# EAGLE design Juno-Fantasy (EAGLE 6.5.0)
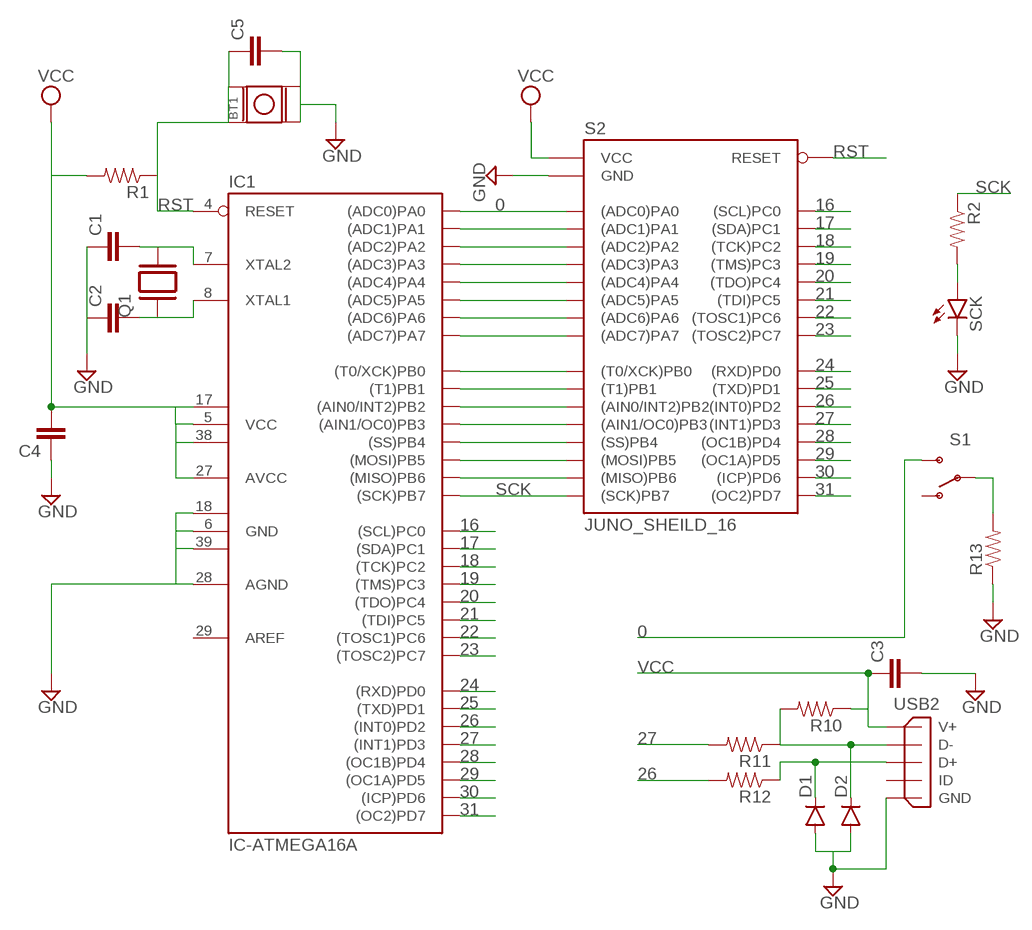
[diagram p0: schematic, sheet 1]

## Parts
BT1  BUTTON-4X4-SMD  [BUT-SMD-4X4]
C1  CAP-SMD-0805  [0805]
C2  CAP-SMD-0805  [0805]
C3  CAP-SMD-0805  [0805]
C4  CAP-SMD-0805  [0805]
C5  CAP-SMD-0805  [0805]
D1  DIODE-SOD-1206  [SOD-1206]
D2  DIODE-SOD-1206  [SOD-1206]
IC1  IC-ATMEGA16A  [TQFP44]
Q1  CRYSTAL-2*6-TH  [CRYSTAL-2*6MM-TH]
R1  RESISTOR-SMD-0805  [0805-R]
R2  RESISTOR-SMD-0805  [0805-R]
R10  RESISTOR-SMD-0805  [0805-R]
R11  RESISTOR-SMD-0805  [0805-R]
R12  RESISTOR-SMD-0805  [0805-R]
R13  RESISTOR-SMD-0805  [0805-R]
S1  SPDT-SMALL-MSK-12C01  [SPDT-SMD]
S2  JUNO_SHEILD_16  [JUNO_SHEILD_16]
SCK  LED-SMD-0805  [LED-0805]
USB2  USB-MICRO  [USB-MICRO]

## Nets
0: IC1.37((ADC0)PA0) S1.1(OFF) S2.A0((ADC0)PA0) S2.A0-((ADC0)PA0)
16: IC1.19((SCL)PC0) S2.C0((SCL)PC0) S2.C0-((SCL)PC0)
17: IC1.20((SDA)PC1) S2.C1((SDA)PC1) S2.C1-((SDA)PC1)
18: IC1.21((TCK)PC2) S2.C2((TCK)PC2) S2.C2-((TCK)PC2)
19: IC1.22((TMS)PC3) S2.C3((TMS)PC3) S2.C3-((TMS)PC3)
20: IC1.23((TDO)PC4) S2.C4((TDO)PC4) S2.C4-((TDO)PC4)
21: IC1.24((TDI)PC5) S2.C5((TDI)PC5) S2.C5-((TDI)PC5)
22: IC1.25((TOSC1)PC6) S2.C6((TOSC1)PC6) S2.C6-((TOSC1)PC6)
23: IC1.26((TOSC2)PC7) S2.C7((TOSC2)PC7) S2.C7-((TOSC2)PC7)
24: IC1.9((RXD)PD0) S2.D0((RXD)PD0) S2.D0-((RXD)PD0)
25: IC1.10((TXD)PD1) S2.D1((TXD)PD1) S2.D1-((TXD)PD1)
26: IC1.11((INT0)PD2) R12.2 S2.D2((INT0)PD2) S2.D2-((INT0)PD2)
27: IC1.12((INT1)PD3) R11.2 S2.D3((INT1)PD3) S2.D3-((INT1)PD3)
28: IC1.13((OC1B)PD4) S2.D4((OC1B)PD4) S2.D4-((OC1B)PD4)
29: IC1.14((OC1A)PD5) S2.D5((OC1A)PD5) S2.D5-((OC1A)PD5)
30: IC1.15((ICP)PD6) S2.D6((ICP)PD6) S2.D6-((ICP)PD6)
31: IC1.16((OC2)PD7) S2.D7((OC2)PD7) S2.D7-((OC2)PD7)
GND: BT1.A0 BT1.A1 C1.1 C2.1 C3.2 C4.1 C5.2 D1.A D2.A IC1.6(GND) IC1.18(GND1) IC1.28(AGND) IC1.39(GND2) R13.1 S2.GND1(GND) S2.GND2(GND) S2.GND3(GND) SCK.C USB2.GND
N$1: C1.2 IC1.7(XTAL2) Q1.P$2
N$2: C2.2 IC1.8(XTAL1) Q1.P$1
N$3: R13.2 S1.2(MID)
N$4: IC1.36((ADC1)PA1) S2.A1((ADC1)PA1) S2.A1-((ADC1)PA1)
N$5: IC1.35((ADC2)PA2) S2.A2((ADC2)PA2) S2.A2-((ADC2)PA2)
N$6: IC1.34((ADC3)PA3) S2.A3((ADC3)PA3) S2.A3-((ADC3)PA3)
N$7: IC1.33((ADC4)PA4) S2.A4((ADC4)PA4) S2.A4-((ADC4)PA4)
N$8: IC1.32((ADC5)PA5) S2.A5((ADC5)PA5) S2.A5-((ADC5)PA5)
N$9: IC1.31((ADC6)PA6) S2.A6((ADC6)PA6) S2.A6-((ADC6)PA6)
N$10: IC1.30((ADC7)PA7) S2.A7((ADC7)PA7) S2.A7-((ADC7)PA7)
N$12: IC1.40((T0/XCK)PB0) S2.B0((T0/XCK)PB0) S2.B0-((T0/XCK)PB0)
N$13: IC1.41((T1)PB1) S2.B1((T1)PB1) S2.B1-((T1)PB1)
N$14: IC1.42((AIN0/INT2)PB2) S2.B2((AIN0/INT2)PB2) S2.B2-((AIN0/INT2)PB2)
N$15: IC1.43((AIN1/OC0)PB3) S2.B3((AIN1/OC0)PB3) S2.B3-((AIN1/OC0)PB3)
N$16: IC1.44((SS)PB4) S2.B4((SS)PB4) S2.B4-((SS)PB4)
N$17: IC1.1((MOSI)PB5) S2.B5((MOSI)PB5) S2.B5-((MOSI)PB5) S2.MOSI((MOSI)PB5)
N$18: IC1.2((MISO)PB6) S2.B6((MISO)PB6) S2.B6-((MISO)PB6) S2.MISO((MISO)PB6)
N$20: R2.2 SCK.A
N$29: D2.C R10.2 R11.1 USB2.D-
N$30: D1.C R12.1 USB2.D+
RST: BT1.B1(B0) BT1.B2(B1) C5.1 IC1.4(RESET) R1.1 S2.RST1(RESET) S2.RST2(RESET)
SCK: IC1.3((SCK)PB7) R2.1 S2.B7((SCK)PB7) S2.B7-((SCK)PB7) S2.SCK((SCK)PB7)
VCC: C3.1 C4.2 IC1.5(VCC) IC1.17(VCC1) IC1.27(AVCC) IC1.38(VCC2) R1.2 R10.1 S2.VCC1(VCC) S2.VCC2(VCC) S2.VCC3(VCC) USB2.V+
Unconnected: S1.3(ON) USB2.ID

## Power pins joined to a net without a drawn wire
AREF: IC1.29(AREF)

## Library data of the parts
BT1 = My Eagle lbr:BUTTON
C1-C5 = My Eagle lbr:CAP-SMD
D1 D2 = My Eagle lbr:DIODE: Diode
IC1 = My Eagle lbr:IC-ATMEGA16: MICROCONTROLLER 16 Kbytes FLASH 1 kbytes SRAM 512 bytes EEPROM USART 8-channel 10 bit ADC
Q1 = My Eagle lbr:CRYSTAL: CRYSTAL
R1 R2 R10-R13 = My Eagle lbr:RESISTOR-SMD
S1 = My Eagle lbr:SPDT-SMALL: SPDT-Switch
S2 = My Eagle lbr:JUNO_SHEILD_16
SCK = My Eagle lbr:LED-SMD
USB2 = My Eagle lbr:USB

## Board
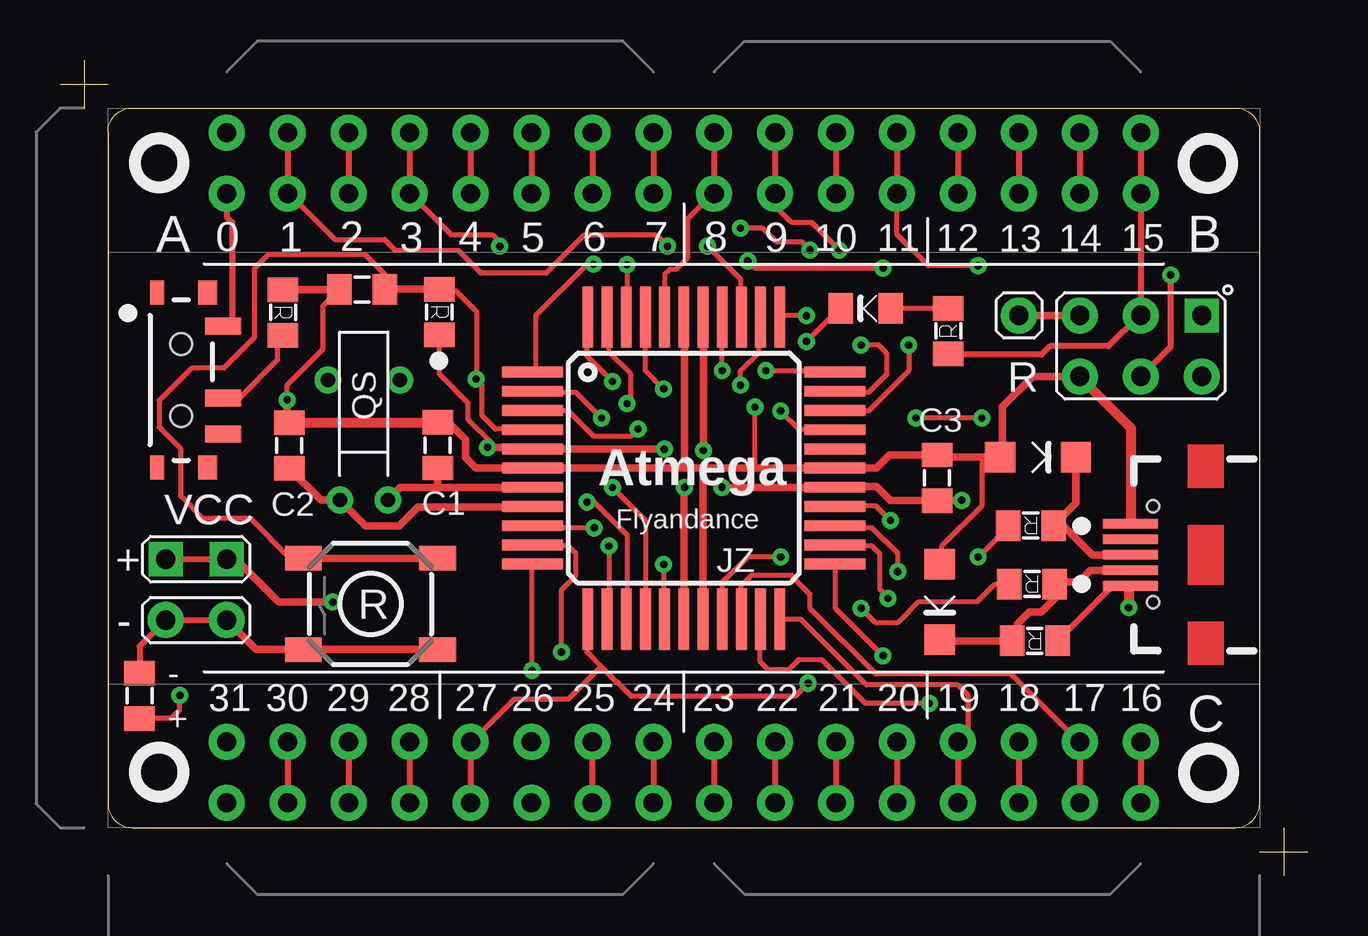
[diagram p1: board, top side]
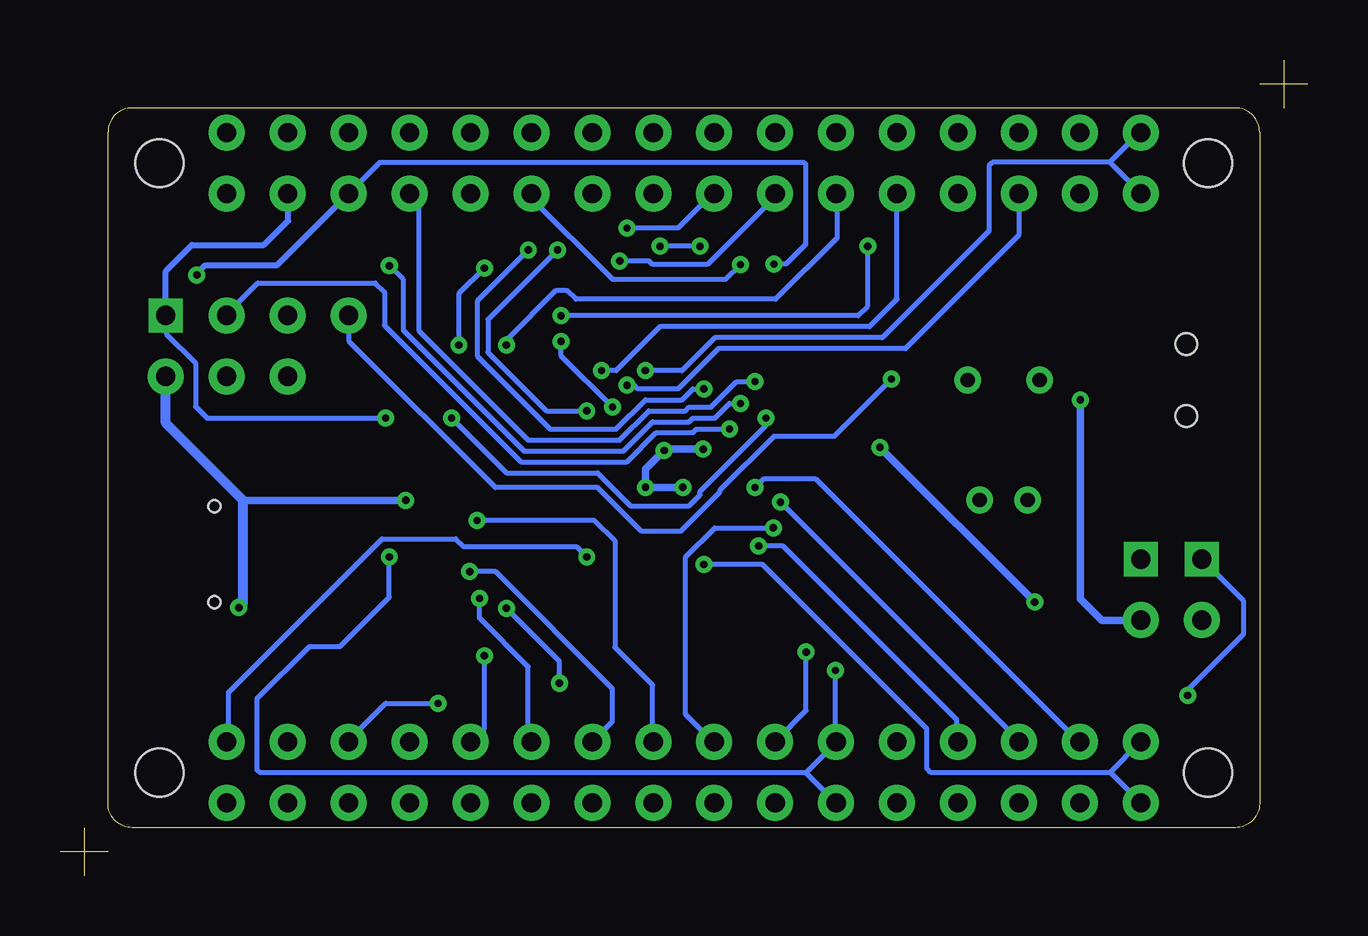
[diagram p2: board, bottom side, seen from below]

Size 52 x 34 mm. Coordinates in mm from the lower left corner, seen from the top.
Outline: 0,33 2,33
Outline: 1,34 1,32
Outline: 50,1 52,1
Outline: 51,2 51,0
Outline: 2,3 arc90 3,2 49,2 arc90 50,3 50,31 arc90 49,32 3,32 arc90 2,31 2,3
Copper layers (1*16): Top 0.035mm / dielectric 1.5mm / Bottom 0.035mm
Design rules "6mm-15mil *": minimum track width 8mil, minimum drill 0.3mm, track to track 6mil, track to pad 15mil, pad to pad 15mil, via to via 10mil, smd to smd 6mil, copper to edge 10mil, drill to drill 6mil, minimum pad ring 10mil, minimum via ring 8mil, stop-mask expansion 1mil, vias tented up to drill 0.4mm, thermal gap 10mil

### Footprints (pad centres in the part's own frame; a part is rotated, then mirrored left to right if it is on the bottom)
BUT-SMD-4X4 = smd 1.524 x 1.016: A0 -2.794,1.905; A1 2.794,1.905; B1 -2.794,-1.905; B2 2.794,-1.905
0805 = smd 1.016 x 1.27: 1 -0.95,0; 2 0.95,0
SOD-1206 = smd 1.27 x 1.27: A 1.575,0; C -1.575,0
TQFP44 = smd 2.55 x 0.45: 1 -6.3,4; 2 -6.3,3.2; 3 -6.3,2.4; 4 -6.3,1.6; 5 -6.3,0.8; 6 -6.3,0; 7 -6.3,-0.8; 8 -6.3,-1.6; 9 -6.3,-2.4; 10 -6.3,-3.2; 11 -6.3,-4; 23 6.3,-4; 24 6.3,-3.2; 25 6.3,-2.4; 26 6.3,-1.6; 27 6.3,-0.8; 28 6.3,0; 29 6.3,0.8; 30 6.3,1.6; 31 6.3,2.4; 32 6.3,3.2; 33 6.3,4 | smd 0.45 x 2.55: 12 -4,-6.3; 13 -3.2,-6.3; 14 -2.4,-6.3; 15 -1.6,-6.3; 16 -0.8,-6.3; 17 0,-6.3; 18 0.8,-6.3; 19 1.6,-6.3; 20 2.4,-6.3; 21 3.2,-6.3; 22 4,-6.3; 34 4,6.3; 35 3.2,6.3; 36 2.4,6.3; 37 1.6,6.3; 38 0.8,6.3; 39 0,6.3; 40 -0.8,6.3; 41 -1.6,6.3; 42 -2.4,6.3; 43 -3.2,6.3; 44 -4,6.3
CRYSTAL-2*6MM-TH = drill 0.6 pad 1: NC1 -1.5,5; NC2 1.5,5 | drill 0.6: P$1 -1,0; P$2 1,0
0805-R = smd 1.016 x 1.27: 1 -0.95,0; 2 0.95,0
SPDT-SMD = smd 1.5 x 0.7: 1 1.75,2.25; 2 1.75,-0.75; 3 1.75,-2.25 | smd 0.6 x 1: GND5 -1,-3.65; GND7 -1,3.65 | smd 0.8 x 1: GND6 1.1,-3.65; GND8 1.1,3.65 | hole 0.9: 0,-1.5; 0,1.5
JUNO_SHEILD_16 = drill 0.8 pad 1.5: A0 -19.05,13.97; A0- -19.05,11.43; A1 -16.51,13.97; A1- -16.51,11.43; A2 -13.97,13.97; A2- -13.97,11.43; A3 -11.43,13.97; A3- -11.43,11.43; A4 -8.89,13.97; A4- -8.89,11.43; A5 -6.35,13.97; A5- -6.35,11.43; A6 -3.81,13.97; A6- -3.81,11.43; A7 -1.27,13.97; A7- -1.27,11.43; B0 1.27,13.97; B0- 1.27,11.43; B1 3.81,13.97; B1- 3.81,11.43; B2 6.35,13.97; B2- 6.35,11.43; B3 8.89,13.97; B3- 8.89,11.43; B4 11.43,13.97; B4- 11.43,11.43; B5 13.97,13.97; B5- 13.97,11.43; B6 16.51,13.97; B6- 16.51,11.43; B7 19.05,13.97; B7- 19.05,11.43; C0 19.05,-13.97; C0- 19.05,-11.43; C1 16.51,-13.97; C1- 16.51,-11.43; C2 13.97,-13.97; C2- 13.97,-11.43; C3 11.43,-13.97; C3- 11.43,-11.43; C4 8.89,-13.97; C4- 8.89,-11.43; C5 6.35,-13.97; C5- 6.35,-11.43; C6 3.81,-13.97; C6- 3.81,-11.43; C7 1.27,-13.97; C7- 1.27,-11.43; D0 -1.27,-13.97; D0- -1.27,-11.43; D1 -3.81,-13.97; D1- -3.81,-11.43; D2 -6.35,-13.97; D2- -6.35,-11.43; D3 -8.89,-13.97; D3- -8.89,-11.43; D4 -11.43,-13.97; D4- -11.43,-11.43; D5 -13.97,-13.97; D5- -13.97,-11.43; D6 -16.51,-13.97; D6- -16.51,-11.43; D7 -19.05,-13.97; D7- -19.05,-11.43; GND1 -21.59,-6.35; GND2 -19.05,-6.35; GND3 16.51,3.81; MOSI 19.05,3.81; RST1 16.51,6.35; RST2 13.97,6.35; SCK 19.05,6.35; VCC3 21.59,3.81 | drill 0.8 pad 1.422 square: MISO 21.59,6.35; VCC1 -21.59,-3.81; VCC2 -19.05,-3.81 | hole 2: -21.86,12.7; 21.86,12.7; 21.86,-12.7; -21.86,-12.7
LED-0805 = smd 1.016 x 1.27: A -1.052,0; C 1.026,0
USB-MICRO = smd 2.3 x 0.4: D+ 1.65,0.016; D- 1.65,0.666; GND 1.65,-1.284; ID 1.65,-0.634; V+ 1.65,1.316 | hole 0.5: 0.708,2; 0.708,-2

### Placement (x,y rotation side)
BT1  12.94,11.32 180 top
C1  15.74,17.94 270 top
C2  9.56,17.93 270 top
C3  36.56,16.58 90 top
C4  3.32,7.5 270 top
C5  12.59,24.43 180 top
D1  40.77,17.44 180 top
D2  36.67,11.4 90 top
IC1  26,16.98 0 top
Q1  12.66,15.66 0 top
R1  15.81,23.49 270 top
R2  37.03,22.7 90 top
R10  40.63,9.78 180 top
R11  40.51,12.15 180 top
R12  40.46,14.59 180 top
R13  9.3,23.47 270 top
S1  5.05,20.66 0 top
S2  26,17 0 top
SCK  33.57,23.64 180 top
USB2  46.27,13.39 180 top

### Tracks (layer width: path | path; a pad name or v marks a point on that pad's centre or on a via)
0  (via drill 0.3)
  Top 0.203: v27.6,21.05 27.6,23.18 IC1.37
  Top 0.254: S2.A0- 6.95,27.45 7.18,27.22 7.18,22.91 S1.1
  Top 0.305: S1.1
  Bottom 0.203: v27.6,21.05 26.08,21.05 24.71,22.42 17.72,22.42 13.28,26.87 13.28,29.58 13.12,29.74 8.25,29.74 | 8.25,29.74 7.03,30.96 S2.A0 | 8.25,29.74 S2.A0-
16  (via drill 0.3)
  Top 0.203: v30.04,13.28 28.67,13.28 27.6,12.21 IC1.19
  Top 0.254: S2.C0- S2.C0
  Bottom 0.203: S2.C0- 44.98,5.66 44.98,7.64 38.58,14.04 35.5,14.04 35.17,13.71 30.47,13.71 v30.04,13.28
17
  Top 0.203: IC1.20 28.36,10.69 28.36,12.06 28.82,12.52 30.5,12.52 30.5,12.49 31.26,11.73 31.26,11.14 34,8.4 39.64,8.4 42.39,5.66 S2.C1-
  Top 0.254: S2.C1- S2.C1
18  (via drill 0.3)
  Top 0.203: 29.28,10.53 IC1.21 29.18,10.66 29.18,8.93 29.53,8.58 30.37,8.58 30.78,8.98 31.77,8.98 33.57,7.18 v36.24,7.18
  Top 0.254: S2.C2- S2.C2
  Bottom 0.203: v36.24,7.18 38.42,7.18 39.95,5.66 S2.C2-
19
  Top 0.203: 30.04,10.53 IC1.22 30.88,10.69 33.62,7.94 37.43,7.94 37.84,7.54 37.84,5.98 S2.C3- 37.36,5.66
  Top 0.254: S2.C3- S2.C3
20  (via drill 0.3)
  Top 0.203: v34.31,9.16 32.33,11.14 32.33,12.97 IC1.23
  Top 0.254: S2.C4- S2.C4
  Bottom 0.203: v34.31,9.16 34.31,6.12 34.77,5.66 S2.C4-
21  (via drill 0.3)
  Top 0.203: IC1.24 32.33,13.73 33.85,13.73 34.16,13.43 34.16,11.96 34.51,11.6 v34.51,11.55
  Top 0.254: S2.C5- S2.C5
  Bottom 0.203: S2.C5- 32.48,5.66 32.48,8.71 34.51,10.74 v34.51,11.55
22  (via drill 0.3)
  Top 0.203: v34.92,12.67 34.92,13.43 33.85,14.5 32.33,14.5 IC1.25
  Top 0.254: S2.C6- S2.C6
  Bottom 0.203: v34.92,12.67 33.85,12.67 28.98,7.79 28.98,6.42 29.74,5.66 S2.C6-
23  (via drill 0.3)
  Top 0.203: v34.61,14.8 34,15.41 32.33,15.41 IC1.26
  Top 0.254: S2.C7- S2.C7
  Bottom 0.203: v34.61,14.8 29.71,14.8 28.87,13.96 28.87,9.52 27.3,7.94 27.3,5.66 S2.C7-
24  (via drill 0.3)
  Top 0.203: v22.27,14.5 19.83,14.5 IC1.9
  Top 0.254: S2.D0- S2.D0
  Bottom 0.203: v22.27,14.5 24.71,14.5 25.93,13.28 25.93,6.72 24.86,5.66 S2.D0-
25  (via drill 0.3)
  Top 0.203: v20.9,9.32 20.9,11.91 21.51,12.52 21.51,13.43 21.2,13.73 19.83,13.73 IC1.10
  Top 0.254: S2.D1 S2.D1-
  Bottom 0.203: v20.9,9.32 20.9,6.88 22.12,5.66 S2.D1-
26  (via drill 0.3)
  Top 0.203: v38.27,13.28 39.49,14.5 R12.2 | v19.68,8.55 19.68,12.97 IC1.11
  Bottom 0.203: v38.27,13.28 38.27,11.6 40.33,9.54 41.6,9.54 43.78,7.38 43.78,4.39 43.66,4.29 20.9,4.29 | 20.9,4.29 19.68,5.5 S2.D2- 19.68,5.66 v19.68,8.55 | S2.D2 20.9,4.28 20.9,4.29
27  (via drill 0.3)
  Top 0.203: 22.56,8.72 21.96,9.32 21.96,10.53 IC1.12 | 22.56,8.72 23.79,7.49 30.65,7.49 v31.18,8.02 | 39.49,12.06 R11.2 38.98,12.15 38.25,11.42 35.81,11.42 34.94,10.56 33.98,10.56 v33.39,11.14 | S2.D3- 17.24,5.66 18.94,7.36 21.2,7.36 22.56,8.72
  Top 0.254: S2.D3- S2.D3
  Bottom 0.203: v31.18,8.02 31.18,8.93 v33.39,11.14
28  (via drill 0.3)
  Top 0.203: v22.88,13.73 22.88,10.69 IC1.13
  Top 0.254: S2.D4- S2.D4
  Bottom 0.203: S2.D4- 14.65,5.5 14.62,5.53 14.62,6.5 21.86,13.73 v22.88,13.73
29  (via drill 0.3)
  Top 0.203: v21.96,15.56 22.27,15.56 23.64,14.19 23.64,10.69 IC1.14
  Top 0.254: S2.D5- S2.D5
  Bottom 0.203: v21.96,15.56 12.06,5.66 S2.D5-
30  (via drill 0.3)
  Top 0.203: v23.03,16.17 24.4,14.8 IC1.15
  Top 0.254: S2.D6- S2.D6
  Bottom 0.203: S2.D6- 9.62,5.66 20.49,16.53 22.68,16.53 v23.03,16.17
31  (via drill 0.3)
  Top 0.203: v25.16,12.97 25.16,10.69 IC1.16
  Bottom 0.203: v25.16,12.97 22.73,12.97 15.87,6.12 15.87,4.46 15.69,4.29 8.25,4.29 | 8.25,4.29 7.03,5.5 S2.D7- | S2.D7 8.21,4.29 8.25,4.29
GND  (via drill 0.3)
  Top 0.203: v31.11,22.27 32.48,23.64 SCK.C | 28.98,16.98 v28.98,19.53 | 38.42,17.44 38.42,15.41 36.75,13.73 36.75,13.12 D2.A | v9.47,19.83 9.47,20.44 10.97,21.94 10.97,23.75 C5.2
  Top 0.254: S2.GND2 S2.GND1 3.32,9.56 C4.1
  Top 0.305: C1.1 | C1.1 16.17,18.89 16.22,18.94 16.22,19.07 16.02,18.87 15.46,18.87 | BT1.A0 BT1.A1 8.18,9.42 S2.GND2 | 26.03,16.98 IC1.6 17.34,16.98 16.91,17.42 16.91,18.18 16.2,18.89 C1.1 | 26.03,16.98 26.8,16.98 | 26.8,16.98 28.98,16.98 IC1.28 32.35,16.94 33.01,16.94 33.06,16.99 34.03,16.99 34.58,17.53 C3.2 36.65,17.44 38.42,17.44 D1.A 39.29,17.54 39.29,19.55 40.55,20.81 S2.GND3 | IC1.39 25.98,23.29 26.03,23.23 26.03,16.98 | C2.1 9.47,18.97 v9.47,19.83 | R13.1 C5.2 | C1.1 | IC1.18 26.8,16.98
  Top 0.406: C2.1 C1.1 | USB2.GND 44.65,14.7 44.65,18.64 42.51,20.77 S2.GND3
  Bottom 0.203: v31.11,22.27 31.11,21.66 v28.98,19.53
  Bottom 0.305: v9.47,19.83 9.47,11.53 8.58,10.64 6.96,10.64 S2.GND2
N$1
  Top 0.305: IC1.7 15.64,16.19 | 15.64,16.19 14.19,16.19 Q1.P$2 | C1.2 15.74,16.29 15.64,16.19
N$2
  Top 0.305: IC1.8 19.55,15.38 19.55,15.36 14.93,15.36 14.14,14.57 12.74,14.57 Q1.P$1 10.88,15.66 C2.2
N$3
  Top 0.203: R13.2 9.16,22.42 9.06,22.32 9.06,21.48 7.49,19.91 S1.2 6.72,19.98
  Top 0.254: 9.3,22.41 R13.2
N$4  (via drill 0.3)
  Top 0.203: v26.99,26.23 28.36,24.86 28.36,23.34 IC1.36 | S2.A1- 9.62,28.36 11.47,26.51 13.53,26.51 13.99,26.05 16.61,26.05 17.55,25.11 20.26,25.11 21.84,26.69 24.86,26.69 v25.32,26.23
  Top 0.254: S2.A1 S2.A1-
  Bottom 0.203: v25.32,26.23 v26.99,26.23
N$5  (via drill 0.3)
  Top 0.203: v28.36,20.44 28.36,21.05 29.13,21.81 29.13,23.18 IC1.35
  Top 0.254: S2.A2 S2.A2-
  Bottom 0.203: v28.36,20.44 28.06,20.44 27.91,20.29 26.23,20.29 24.55,21.96 16.76,21.96 12.03,26.69 12.03,28.34 | 12.06,28.36 S2.A2-
  Bottom 0.254: 12.06,28.36 12.03,28.34
N$6  (via drill 0.3)
  Top 0.203: v31.11,23.34 30.04,23.34 IC1.34 | S2.A3- 14.65,28.36 16.3,26.71 18.03,26.71 18.33,26.41 v18.33,26.23
  Top 0.254: S2.A3 S2.A3-
  Bottom 0.203: v31.11,23.34 18.74,23.34 18.33,23.74 v18.33,26.23
N$7  (via drill 0.3)
  Top 0.203: v29.43,21.05 32.17,21.05 IC1.33
  Top 0.254: S2.A4 S2.A4-
  Bottom 0.203: v29.43,21.05 28.82,21.05 26.99,22.88 18.26,22.88 17.11,24.02 S2.A4-
N$8  (via drill 0.3)
  Top 0.203: IC1.32 32.33,20.14 33.7,20.14 34.46,20.9 34.46,21.76 34.11,22.12 v33.39,22.12
  Top 0.254: S2.A5 S2.A5-
  Bottom 0.203: 19.68,28.36 S2.A5- 19.6,28.38 19.6,26.59 22.17,24.02 30.5,24.02 30.85,24.38 31.34,24.38 33.39,22.32 v33.39,22.12
N$9  (via drill 0.3)
  Top 0.203: v35.38,22.12 35.38,21.05 33.7,19.37 32.33,19.37 IC1.31 | v34.31,25.32 28.98,25.32 v28.67,25.62
  Top 0.254: S2.A6 S2.A6-
  Bottom 0.203: v35.38,22.12 35.38,24.25 v34.31,25.32 | v28.67,25.62 27.45,25.62 27.3,25.47 25.01,25.47 22.12,28.36 S2.A6-
N$10  (via drill 0.3)
  Top 0.203: v30.04,19.37 30.8,18.61 32.17,18.61 IC1.30 | v31.26,26.08 30.93,26.41 29.86,26.41 29.28,26.99 v28.36,26.99
  Top 0.254: S2.A7 S2.A7-
  Bottom 0.203: v30.04,19.37 31.72,19.37 34.16,21.81 34.16,23.18 v31.26,26.08 | v28.36,26.99 26.23,26.99 24.86,28.36 S2.A7-
N$11
  Top 0: 0,33 2,33
N$12
  Top 0.203: 25.16,23.34 IC1.40 25.2,25.05 25.42,25.27 25.67,25.27 26.16,25.75 26.16,27.38 27.15,28.36 S2.B0-
  Top 0.254: S2.B0 S2.B0-
N$13  (via drill 0.3)
  Top 0.203: v25.16,20.29 24.4,21.05 24.4,23.18 IC1.41 | 29.89,28.67 S2.B1- 29.81,27.91 30.5,27.22 31.34,27.22 v32.48,26.08
  Top 0.254: S2.B1 S2.B1-
  Bottom 0.203: v25.16,20.29 25.62,20.29 26.08,19.83 27.6,19.83 28.82,18.61 31.57,18.61 34.61,21.66 34.61,23.95 v32.48,26.08
N$14  (via drill 0.3)
  Top 0.203: v23.64,25.47 23.64,23.34 IC1.42
  Top 0.254: S2.B2 S2.B2-
  Bottom 0.203: S2.B2- 32.48,28.36 28.98,24.86 24.25,24.86 v23.64,25.47
N$15  (via drill 0.3)
  Top 0.203: v23.64,19.68 23.79,19.83 23.79,20.9 22.88,21.81 22.88,23.18 IC1.43 | v38.27,25.42 36.19,25.42 34.89,26.71 S2.B3-
  Top 0.254: S2.B3 S2.B3-
  Bottom 0.203: v23.64,19.68 24.1,19.68 24.71,19.07 25.62,19.07 25.77,18.92 27.3,18.92 28.52,17.7 32.66,17.7 37.69,22.73 37.69,24.84 v38.27,25.42 | 34.92,30.96 S2.B3
N$16  (via drill 0.3)
  Top 0.203: v23.03,20.59 21.96,21.66 21.96,23.18 IC1.44
  Top 0.254: S2.B4 S2.B4-
  Bottom 0.203: v23.03,20.59 23.79,20.59 24.86,19.53 25.77,19.53 25.93,19.37 27.45,19.37 28.67,18.15 32.48,18.15 37.05,22.73 37.05,28.06 37.36,28.36 S2.B4-
N$17  (via drill 0.3)
  Top 0.203: IC1.1 19.83,21.05 19.83,23.34 21.99,25.5 v22.24,25.5 | 39.95,28.36 S2.B5-
  Top 0.254: S2.B5 S2.B5- | v46.3,25.04 46.3,22.04 46.28,22.04 S2.MOSI
  Bottom 0.203: S2.B5- 38.66,29.74 21,29.74 20.92,29.66 20.92,26.31 21.74,25.5 v22.24,25.5 | v46.3,25.04 46.3,25.09
  Bottom 0.254: S2.B5- 42.96,25.44 45.94,25.44 46.3,25.09
N$18  (via drill 0.3)
  Top 0.203: v22.57,19.07 21.51,20.14 19.83,20.14 IC1.2 | v38.42,19.07 v35.68,19.07
  Top 0.254: S2.B6 S2.B6-
  Bottom 0.203: v22.57,19.07 22.57,18.76 25.32,16.02 25.32,15.87 25.77,15.41 28.21,15.41 29.58,16.78 33.39,16.78 v35.68,19.07 | v38.42,19.07 45.87,19.07 46.35,19.55 46.35,21.36 47.57,22.57 47.57,23.34 S2.MISO
  Bottom 0.254: S2.MISO 47.59,25.19 46.5,26.28 43.5,26.28 42.49,27.3 42.49,28.41 S2.B6-
N$19
  Top 0: 1,34 1,32
N$20
  Top 0.203: SCK.A 36.9,23.64 R2.2
N$21
  Bottom 0: 0,33 2,33
N$22
  Bottom 0: 1,34 1,32
N$23
  Top 0: 50,1 52,1
N$24
  Top 0: 51,2 51,0
N$25
  Bottom 0: 50,1 52,1
N$26
  Bottom 0: 51,2 51,0
N$29
  Top 0.305: D2.C 36.71,9.78 R10.2 39.9,10 39.9,10.48 40.41,10.99 40.91,10.99 41.47,11.54 R11.1 41.55,12.24 42.46,12.24 42.95,12.72 USB2.D-
N$30
  Top 0.305: D1.C 42.34,15.52 R12.1 41.81,14.59 43.03,13.37 USB2.D+
RST  (via drill 0.3)
  Top 0.203: R1.1 15.87,24.4 16.48,24.4 17.37,23.51 17.37,20.72 v17.34,20.69 17.6,20.44 17.6,19.17 18.15,18.61 19.68,18.61 IC1.4 | 10.08,13.28 BT1.B2 | 13.43,24.55 C5.1 13.54,25.05 12.72,25.88 8.68,25.88 8.1,25.29 8.1,22.42 6.83,21.15 5.48,21.15 4.13,19.8 4.13,18.69 5.02,17.8 5.02,15.82 5.94,14.9 7.92,14.9 9.59,13.23 10.66,13.23
  Top 0.305: BT1.B2 10.66,13.23 BT1.B1 | C5.1 13.25,24.43 13.26,24.44 R1.1 | S2.RST1 S2.RST2
  Bottom 0.203: S2.RST2 39.95,23.34 39.95,22.27 33.85,16.17 29.58,16.17 27.76,14.34 26.13,14.34 24.5,15.97 24.5,16.05 22.24,18.31 19.73,18.31 v17.34,20.69
SCK  (via drill 0.3)
  Top 0.203: v24.1,18.61 23.79,18.31 22.27,18.31 21.2,19.37 19.83,19.37 IC1.3
  Top 0.254: S2.B7 S2.B7- S2.SCK 44.99,23.35 43.71,22.07 41.27,22.07 40.91,21.71 37.07,21.71 R2.1
  Bottom 0.203: v24.1,18.61 25.47,18.61 25.62,18.46 27.15,18.46 28.36,17.24 32.78,17.24 38.47,22.93 38.47,24.33 38.85,24.71 43.76,24.71 44.98,23.49 S2.SCK
VCC  (via drill 0.3)
  Top 0.203: 15.87,22.42 R1.2 15.81,20.9 17.01,19.7 17.01,18.99 18,18 18,17.85 | v5,7.51 4.97,7.49 4.97,6.88 4.64,6.54 C4.2
  Top 0.254: USB2.V+ 43.87,12.07 R10.1 | S2.VCC1 S2.VCC2
  Top 0.305: 36.55,15.64 C3.1 | C3.1 37.58,15.63 v37.59,15.64 | v27.59,16.19 IC1.27 32.34,16.22 34.03,16.22 34.62,15.63 C3.1 | v26.82,17.72 26.82,23.27 IC1.38 | S2.VCC2 6.99,13.15 7.36,13.15 9.11,11.4 v11.37,11.4 | v26.04,16.19 26,16.15 26,10.08 | 26,10.08 | 26,10.08 IC1.17 | v25.19,17.77 20.25,17.77 20.24,17.79 IC1.5 19.64,17.85 18,17.85 v17.82,17.85 | USB2.V+ 44.55,12
  Top 0.406: 44.55,12 v44.55,11.17
  Bottom 0.203: S2.VCC1 2.69,11.47 2.69,10.05 5,7.74 v5,7.51
  Bottom 0.305: v37.59,15.64 44.37,15.64 | S2.VCC3 | v26.04,16.19 v27.59,16.19 27.59,16.95 v26.82,17.72 26.77,17.77 v25.19,17.77 | v11.37,11.4 v17.82,17.85 | v44.55,11.17 44.37,11.35
  Bottom 0.406: S2.VCC3 47.59,18.87 44.37,15.64 44.37,11.35

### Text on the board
tPlace: A | B | R | QS | Atmega | VCC | Flyandance | JZ | R | - | + | C
203bmp: C:/Eagles/PCB-Images/Cover_back_1.0165.bmp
